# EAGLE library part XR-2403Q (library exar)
Enhanced MNP-5 modem MICROCONTROLLER
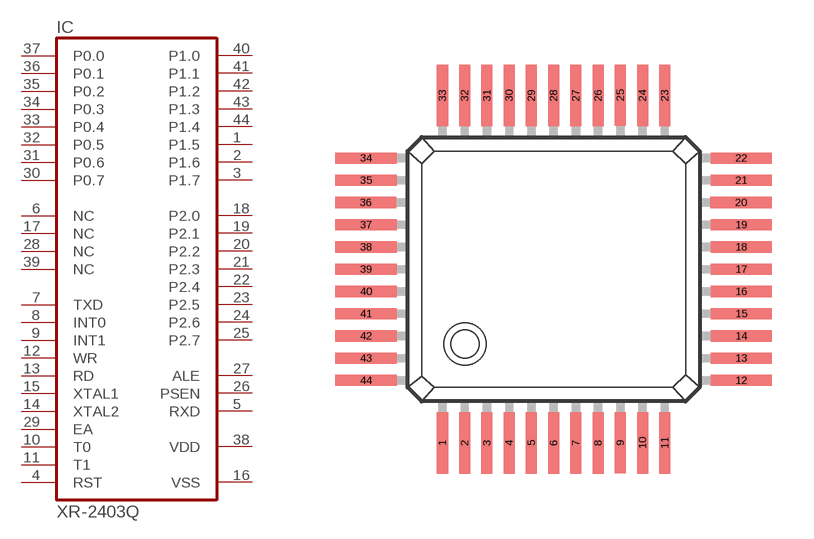
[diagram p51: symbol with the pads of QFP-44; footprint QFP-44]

Designator prefix IC

## XR-2403Q (OC_FARNELL: unknown; OC_NEWARK: unknown)  [QFP-44]
1  P1.5
2  P1.6
3  P1.7
4  RST  in
5  RXD  out
6  NC  nc
7  TXD  in
8  INT0  in
9  INT1  in
10  T0  in
11  T1  in
12  WR  in
13  RD  in
14  XTAL2  in
15  XTAL1  in
16  VSS  pwr
17  NC  nc
18  P2.0
19  P2.1
20  P2.2
21  P2.3
22  P2.4
23  P2.5
24  P2.6
25  P2.7
26  PSEN  out
27  ALE  out
28  NC  nc
29  EA  in
30  P0.7
31  P0.6
32  P0.5
33  P0.4
34  P0.3
35  P0.2
36  P0.1
37  P0.0
38  VDD  pwr
39  NC  nc
40  P1.0
41  P1.1
42  P1.2
43  P1.3
44  P1.4

## Footprint QFP-44 (pad centres in mm)
Quad Flat Package
smd 0.4 x 2.2: 1 -4,-6.25; 2 -3.2,-6.25; 3 -2.4,-6.25; 4 -1.6,-6.25; 5 -0.8,-6.25; 6 0,-6.25; 7 0.8,-6.25; 8 1.6,-6.25; 9 2.4,-6.24; 10 3.2,-6.25; 11 4,-6.25; 23 4,6.25; 24 3.2,6.25; 25 2.4,6.26; 26 1.6,6.25; 27 0.8,6.25; 28 0,6.25; 29 -0.8,6.25; 30 -1.6,6.25; 31 -2.4,6.25; 32 -3.2,6.25; 33 -4,6.25
smd 2.2 x 0.4: 12 6.75,-4; 13 6.75,-3.2; 14 6.75,-2.4; 15 6.75,-1.6; 16 6.75,-0.8; 17 6.75,0; 18 6.75,0.8; 19 6.75,1.6; 20 6.74,2.4; 21 6.75,3.2; 22 6.75,4; 34 -6.75,4; 35 -6.75,3.2; 36 -6.76,2.4; 37 -6.75,1.6; 38 -6.75,0.8; 39 -6.75,0; 40 -6.75,-0.8; 41 -6.75,-1.6; 42 -6.75,-2.4; 43 -6.75,-3.2; 44 -6.75,-4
